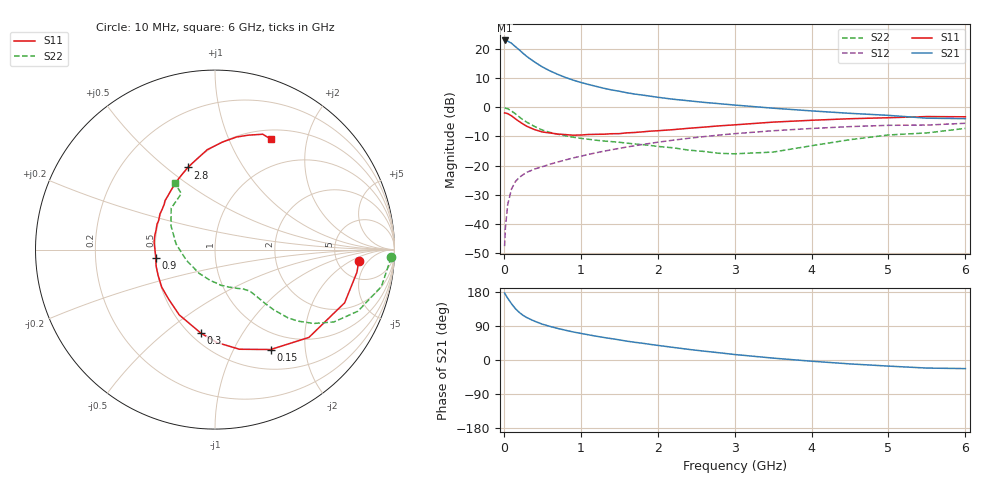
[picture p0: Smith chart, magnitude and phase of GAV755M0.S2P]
! Infineon Technologies  Discrete & RF Semiconductors
! BF775
! Si NPN RF Bipolar Junction Transistor in SOT23
! VCE = 0.75 V  IC = 5 mA
! Common Emitter S-Parameters:  May  1996
# GHz  S  MA  R  50
!  f  S11  S21  S12  S22
! GHz  MAG  ANG  MAG  ANG  MAG  ANG  MAG  ANG
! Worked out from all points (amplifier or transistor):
!   36 points, 10 MHz to 6 GHz, reference 50 ohm
!   highest |S21| = 23.0 dB at 10 MHz (marker M1)
!   |S21| within 3 dB of that: start of sweep to 189.8 MHz
!   unconditionally stable (mu >= 1): 687.3 MHz to end of sweep
!   at 250 MHz: K = 0.52, MSG = 20.9 dB, |S12| = -23.1 dB
!   at 1.4 GHz: K = 1.19, MAG = 7.6 dB, |S12| = -14.6 dB
!   at 6 GHz: K = 1.05, MAG = -0.6 dB, |S12| = -5.5 dB
!   S11 on the Smith chart (normalised r, x): 10 MHz: 8.09, -2.94; 150 MHz: 0.76, -1.42; 300 MHz: 0.56, -0.68; 900 MHz: 0.50, -0.05; 2.8 GHz: 0.50, +0.60; 6 GHz: 0.62, +1.44
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0.01  0.8034 -4.6  14.19 176.8  0.0041 83.2  0.9827 -2.5
0.02  0.8008 -9.1  13.97 173.1  0.0084 85.7  0.9709 -5.1
0.05  0.7808 -22.3  13.84 163.2  0.0213 78.1  0.9498 -12.5
0.1  0.7163 -43.1  12.69 148.3  0.0396 68.7  0.8671 -23.3
0.15  0.6372 -60.9  11.1 135.4  0.0529 60.9  0.7757 -31.3
0.2  0.5717 -76.2  9.794 125.7  0.0623 56.3  0.6869 -36.8
0.25  0.5178 -88.8  8.519 117.8  0.0697 53.2  0.6099 -40.8
0.3  0.4725 -99.5  7.497 111.8  0.0766 51.5  0.5556 -43.1
0.4  0.4148 -118.7  6.038 102.3  0.087 49.8  0.4695 -45.7
0.5  0.3783 -133.0  4.977 94.6  0.0954 49.8  0.4081 -47.1
0.6  0.3633 -144.7  4.247 88.6  0.1054 50.2  0.3715 -47.8
0.7  0.3482 -155.4  3.71 83.3  0.115 50.6  0.3459 -48.5
0.9  0.3328 -172.3  2.954 74.1  0.1351 51.3  0.3074 -49.8
1.1  0.3421 172.9  2.484 66.5  0.1554 51.7  0.283 -52.5
1.3  0.3458 161.9  2.135 59.5  0.1765 50.9  0.2642 -55.6
1.6  0.3652 147.2  1.787 49.7  0.2084 49.3  0.243 -61.9
2.2  0.4145 125.5  1.384 33.3  0.2729 44.1  0.2021 -80.3
2.8  0.4818 108.3  1.159 19.1  0.3349 37.1  0.1623 -110.8
3.5  0.5587 94.4  0.97 5.0  0.3968 27.7  0.1704 -159.8
4.5  0.6389 79.1  0.791 -10.3  0.4675 14.4  0.2787 151.6
5.5  0.6957 67.5  0.653 -21.3  0.4968 0.8  0.3641 121.0
6  0.6897 63.1  0.641 -22.7  0.5335 -2.9  0.4357 121.1
